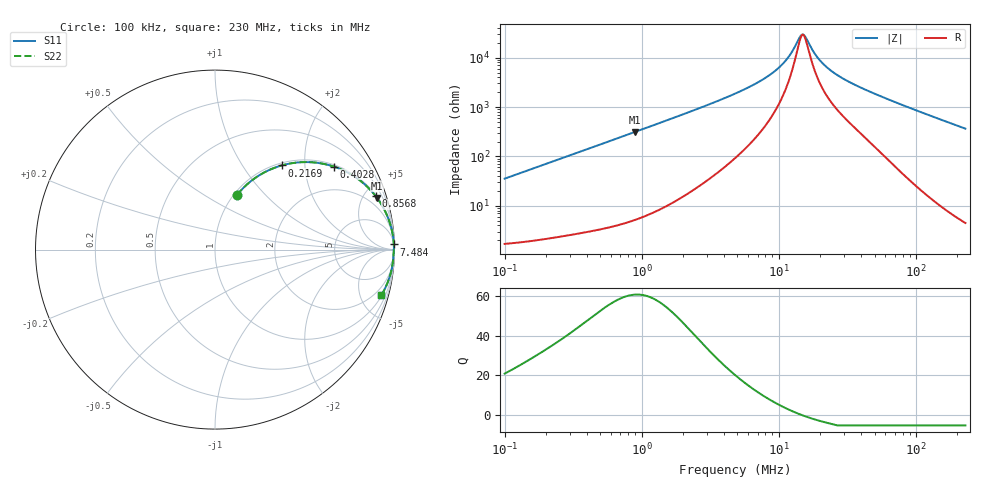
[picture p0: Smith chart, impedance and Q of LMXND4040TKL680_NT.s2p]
! LMXND4040TKL680_NT  S-PARAMETER MODEL  ( Standard Model )
! Model Generated by TAIYO YUDEN Corporation (https://www.yuden.co.jp/en/)
! Version 1.0
! TAIYO YUDEN Control No. 20251120
! Copyright(c) 2025 TAIYO YUDEN CO.,LTD. All Rights Reserved.
! Product Description (link to TY-COMPAS)
! https://ds.yuden.co.jp/TYCOMPAS/or/detail?pn=LMXND4040TKL680MNT&u=M
! Products Name : Inductors
! Characteristics :
!  Inductance : 68 [uH] , SRF(min) : 8.3 [MHz] , DC Resistance(max) : 1.2 [Ohm]
!  Rated Current : Saturation  520 [mA] , Temp Rise  565 [mA] (40 [degC])
!  Case Size : 4.0 x 4.0 / 0.157 x 0.157 [mm/inch] , Thickness : 1.8 / 0.071 [mm/inch]
!  (Conditions: Temperature = 25 [degC] , DC Bias Current = 0 [A])
! External Node Assignments :
!  1  o---GGG---o  2
! GND o---------o GND
! Frequency Range : 0.1MHz  -  229.966873MHz  [ 402 STEP ]
# MHz S RI R 50
! Freq[MHz].  S11 Real  S11 Imag  S21 Real  S21 Imag  S12 Real  S12 Imag  S22 Real  S22 Imag
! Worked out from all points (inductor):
!   401 points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, 100 kHz to 230 MHz, reference 50 ohm
!   read as one part in series: L = 56.2 uH near 103.9 kHz
!   highest Q = 60.5 at 890.6 kHz (marker M1), where L = 55.7 uH
!   self-resonance near 14.73 MHz
!   S11 on the Smith chart (normalised r, x): 100 kHz: 1.03, +0.71; 216.9 kHz: 1.04, +1.53; 402.8 kHz: 1.06, +2.82; 856.8 kHz: 1.10, +6.00; 7.484 MHz: 8, +69; 230 MHz: 1.09, -7.30
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0.1  0.123 0.3054  0.877 -0.3054  0.877 -0.3054  0.123 0.3054
0.147259  0.2213 0.3972  0.7787 -0.3972  0.7787 -0.3972  0.2213 0.3972
0.216854  0.3717 0.469  0.6283 -0.469  0.6283 -0.469  0.3717 0.469
0.365661  0.6191 0.4747  0.3809 -0.4747  0.3809 -0.4747  0.6191 0.4747
0.40281  0.6625 0.4625  0.3375 -0.4625  0.3375 -0.4625  0.6625 0.4625
0.856766  0.896 0.2971  0.104 -0.2971  0.104 -0.2971  0.896 0.2971
0.890575  0.9029 0.288  0.0971 -0.288  0.0971 -0.288  0.9029 0.288
1.337081  0.9534 0.2021  0.0466 -0.2021  0.0466 -0.2021  0.9534 0.2021
4.889189  0.9947 0.0519  0.00535 -0.0519  0.00535 -0.0519  0.9947 0.0519
7.483907  0.9965 0.0285  0.00355 -0.0285  0.00355 -0.0285  0.9965 0.0285
9.259215  0.9968 0.0189  0.00321 -0.0189  0.00321 -0.0189  0.9968 0.0189
10.80955  0.9969 0.0125  0.00314 -0.0125  0.00314 -0.0125  0.9969 0.0125
12.14039  0.9968 0.00799  0.00317 -0.00799  0.00317 -0.00799  0.9968 0.00799
14.17313  0.9967 0.00213  0.0033 -0.00213  0.0033 -0.00213  0.9967 0.00213
14.73242  0.9966 0.000682  0.00336 -0.000682  0.00336 -0.000682  0.9966 0.000682
15.61301  0.9966 -0.00147  0.00345 0.00147  0.00345 0.00147  0.9966 -0.00147
17.53523  0.9963 -0.00577  0.00368 0.00577  0.00368 0.00577  0.9963 -0.00577
20.87128  0.9959 -0.0123  0.00412 0.0123  0.00412 0.0123  0.9959 -0.0123
26.84128  0.9951 -0.022  0.00493 0.022  0.00493 0.022  0.9951 -0.022
37.297  0.9939 -0.0366  0.00609 0.0366  0.00609 0.0366  0.9939 -0.0366
64.11956  0.9909 -0.0704  0.00909 0.0704  0.00909 0.0704  0.9909 -0.0704
229.9669  0.9276 -0.2531  0.0724 0.2531  0.0724 0.2531  0.9276 -0.2531
